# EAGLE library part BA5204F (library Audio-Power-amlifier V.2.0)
3V / 35mW dual power amplifier
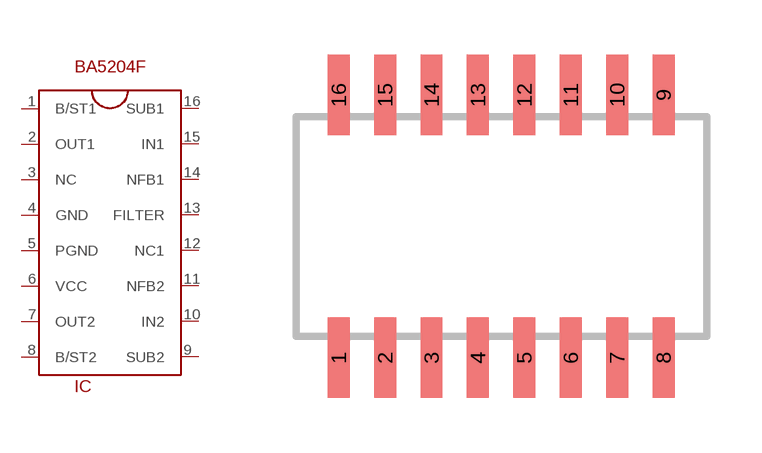
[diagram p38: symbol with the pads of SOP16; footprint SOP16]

Designator prefix IC

## BA5204F  [SOP16]
1  B/ST1
2  OUT1  out
3  NC  nc
4  GND  pwr
5  PGND  pwr
6  VCC  pwr
7  OUT2  out
8  B/ST2
9  SUB2
10  IN2  in
11  NFB2
12  NC1  nc
13  FILTER
14  NFB1
15  IN1  in
16  SUB1

## Footprint SOP16 (pad centres in mm)
smd 0.6 x 2.2: 1 -4.445,-3.6; 2 -3.175,-3.6; 3 -1.905,-3.6; 4 -0.635,-3.6; 5 0.635,-3.6; 6 1.905,-3.6; 7 3.175,-3.6; 8 4.445,-3.6; 9 4.445,3.6; 10 3.175,3.6; 11 1.905,3.6; 12 0.635,3.6; 13 -0.635,3.6; 14 -1.905,3.6; 15 -3.175,3.6; 16 -4.445,3.6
